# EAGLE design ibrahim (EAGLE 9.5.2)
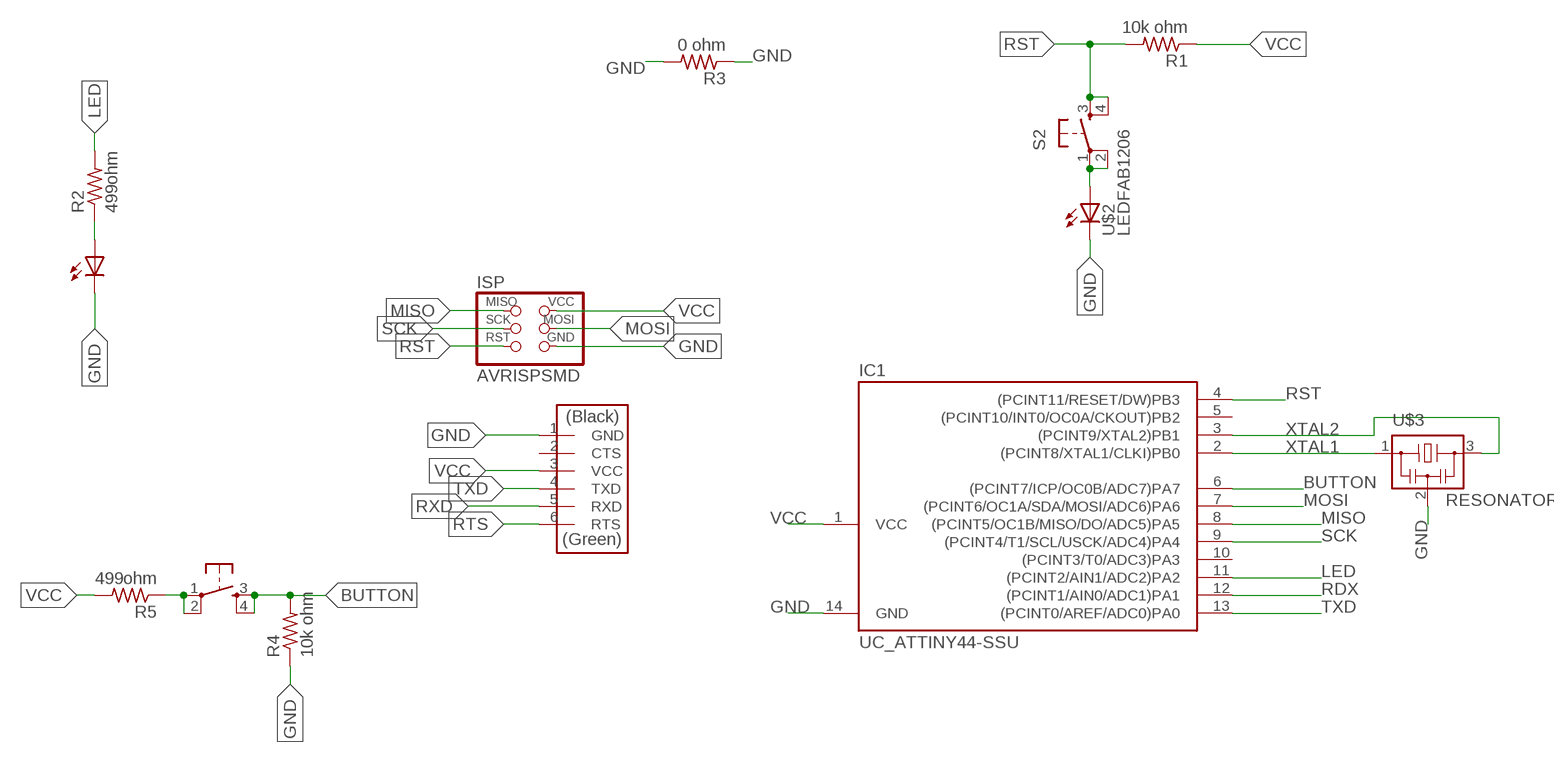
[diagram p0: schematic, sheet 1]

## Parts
IC1  UC_ATTINY44-SSU  [SOIC14]
ISP  AVRISPSMD  [2X03SMD]
R1  10k ohm  R1206FAB  [R1206FAB]
R2  499ohm  R1206FAB  [R1206FAB]
R3  0 ohm  R1206FAB  [R1206FAB]
R4  10k ohm  R1206FAB  [R1206FAB]
R5  499ohm  R1206FAB  [R1206FAB]
S1  6MM_SWITCH6MM_SWITCH  [6MM_SWITCH]
S2  6MM_SWITCH6MM_SWITCH  [6MM_SWITCH]
U$1  FTDI-SMD-HEADER  [1X06SMD]
U$2  LEDFAB1206  [LED1206FAB]
U$3  RESONATOR  [EFOBM]
U$6  LEDFAB1206  [LED1206FAB]

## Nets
BUTTON: IC1.6((PCINT7/ICP/OC0B/ADC7)PA7) R4.2 S1.3(S) S1.4(S1)
GND: IC1.14(GND) ISP.6(GND) R3.1 R3.2 R4.1 U$1.1(GND) U$2.2(C) U$3.2 U$6.2(C)
LED: IC1.11((PCINT2/AIN1/ADC2)PA2) R2.2
MISO: IC1.8((PCINT5/OC1B/MISO/DO/ADC5)PA5) ISP.1(MISO)
MOSI: IC1.7((PCINT6/OC1A/SDA/MOSI/ADC6)PA6) ISP.4(MOSI)
N$1: R2.1 U$6.1(A)
N$2: R5.1 S1.1(P) S1.2(P1)
N$3: S2.1(P) S2.2(P1) U$2.1(A)
RDX: IC1.12((PCINT1/AIN0/ADC1)PA1)
RST: IC1.4((PCINT11/RESET/DW)PB3) ISP.5(RST) R1.2 S2.3(S) S2.4(S1)
RTS: U$1.6(RTS)
RXD: U$1.5(RXD)
SCK: IC1.9((PCINT4/T1/SCL/USCK/ADC4)PA4) ISP.3(SCK)
TXD: IC1.13((PCINT0/AREF/ADC0)PA0) U$1.4(TXD)
VCC: IC1.1(VCC) ISP.2(VCC) R1.1 R5.2 U$1.3(VCC)
XTAL1: IC1.2((PCINT8/XTAL1/CLKI)PB0) U$3.1
XTAL2: IC1.3((PCINT9/XTAL2)PB1) U$3.3
Unconnected: IC1.5((PCINT10/INT0/OC0A/CKOUT)PB2) IC1.10((PCINT3/T0/ADC3)PA3) U$1.2(CTS)

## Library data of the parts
IC1 = fab:UC_ATTINY44
ISP = fab:AVRISP
R1-R5 = fab:R: Resistor (US Symbol)
S1 S2 = fab:6MM_SWITCH: OMRON SWITCH
U$1 = fab:FTDI-SMD-HEADER
U$2 U$6 = fab:LED: LED
U$3 = fab:RESONATOR

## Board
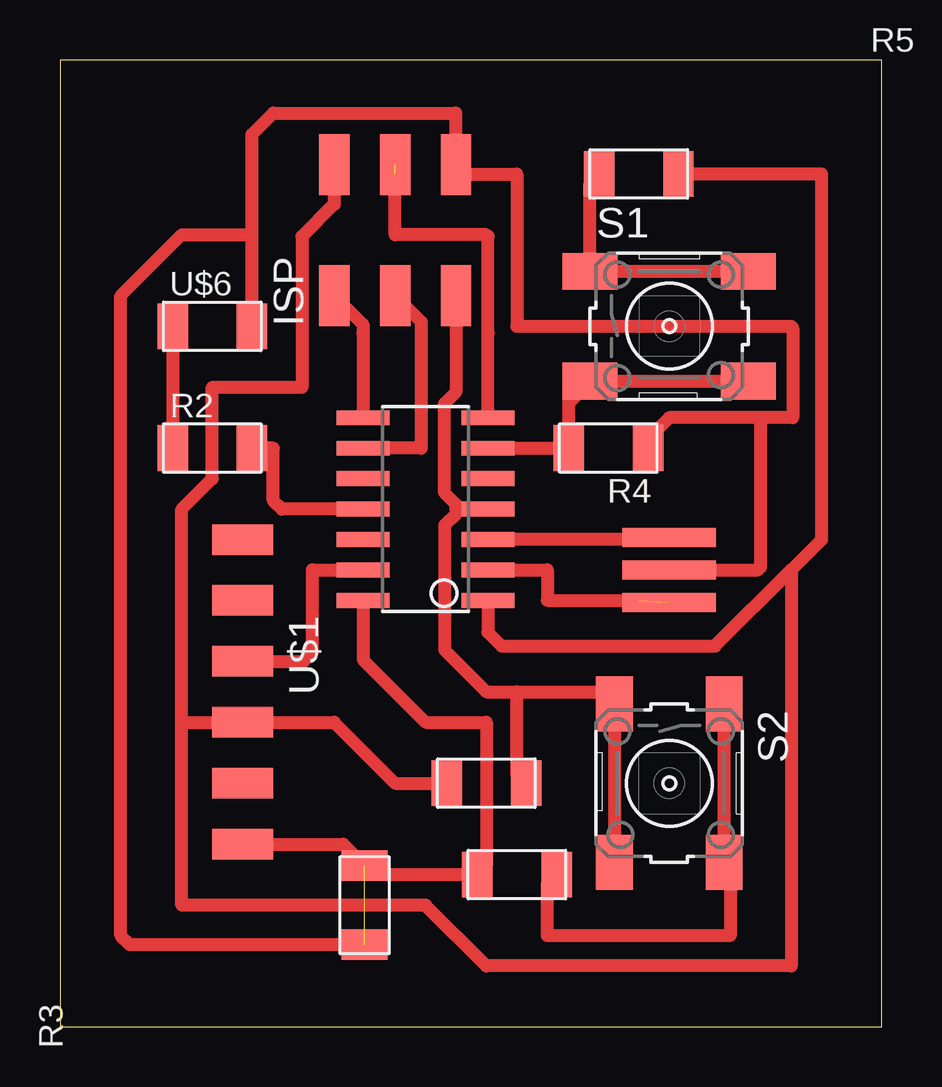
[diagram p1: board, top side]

Size 34.27 x 40.31 mm. Coordinates in mm from the lower left corner, seen from the top.
Outline: 0,0 34.27,0 34.27,40.31 0,40.31 0,0
Copper layers (1*16): Top 0.035mm / dielectric 1.5mm / Bottom 0.035mm
Design rules "default *": minimum track width 0.55mm, minimum drill 0.35mm, track to track 0.43mm, track to pad 0.43mm, pad to pad 0.43mm, via to via 0.43mm, smd to smd 6mil, copper to edge 40mil, drill to drill 6mil, minimum pad ring 10mil, minimum via ring 8mil, stop-mask expansion 4mil, vias tented up to drill 0mil, thermal gap 10mil

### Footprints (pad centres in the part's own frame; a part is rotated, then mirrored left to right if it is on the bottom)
SOIC14 = smd 0.61 x 2.21: 1 -3.81,-2.603; 2 -2.54,-2.603; 3 -1.27,-2.603; 4 0,-2.603; 5 1.27,-2.603; 6 2.54,-2.603; 7 3.81,-2.603; 8 3.81,2.603; 9 2.54,2.603; 10 1.27,2.603; 11 0,2.603; 12 -1.27,2.603; 13 -2.54,2.603; 14 -3.81,2.603
2X03SMD = smd 2.54 x 1.27: 1 -2.54,2.54; 2 2.92,2.54; 3 -2.54,0; 4 2.92,0; 5 -2.54,-2.54; 6 2.92,-2.54
R1206FAB = smd 1.27 x 1.905: 1 -1.651,0; 2 1.651,0
6MM_SWITCH = smd 2.286 x 1.524: 1 -3.302,2.286; 2 3.302,2.286; 3 -3.302,-2.286; 4 3.302,-2.286
1X06SMD = smd 2.54 x 1.27: 1 0,6.35; 2 0,3.81; 3 0,1.27; 4 0,-1.27; 5 0,-3.81; 6 0,-6.35
LED1206FAB = smd 1.27 x 1.905: 1 -1.651,0; 2 1.651,0
EFOBM = smd 0.8 x 3.9: 1 -1.35,0; 2 0,0; 3 1.35,0

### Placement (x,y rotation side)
IC1  15.24,21.59 90 top
ISP  13.97,33.02 90 top
R1  17.78,10.16 0 top
R2  6.35,24.13 0 top
R3  12.7,5.08 90 top
R4  22.86,24.13 180 top
R5  24.13,35.56 0 top
S1  25.4,29.21 0 top
S2  25.4,10.16 270 top
U$1  7.62,13.97 180 top
U$2  19.05,6.35 180 top
U$3  25.4,19.05 90 top
U$6  6.35,29.21 0 top

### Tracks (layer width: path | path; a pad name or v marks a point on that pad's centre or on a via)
BUTTON
  Top 0.55: IC1.6 R4.2 | R4.2 21.59,24.51 | S1.4 S1.3 21.21,26.04 R4.2
GND  (1 unrouted)
  Top 0.55: 29.21,25.4 30.55,25.4 30.55,29.14 30.48,29.21 19.05,29.21 19.05,35.56 16.89,35.56 ISP.6 16.51,38.1 8.89,38.1 8,37.21 8,33.02 | 29.21,25.4 25.4,25.4 24.51,24.51 R4.1 | U$3.2 29.09,19.05 29.21,19.17 29.21,25.4 | 7.62,29.59 U$6.2 8,33.02 | IC1.14 12.64,15.3 15.24,12.7 17.78,12.7 17.78,6.73 U$2.2 13.08,6.35 R3.2 11.81,7.62 U$1.1 | R3.1 2.92,3.43 2.54,3.81 2.54,30.48 5.08,33.02 8,33.02
LED
  Top 0.55: 12.7,21.59 IC1.11 9.25,21.59 8.89,21.95 8.89,24.13 R2.2
MISO
  Top 0.55: ISP.1 12.63,29.28 12.63,28.92 12.64,28.91 IC1.8
MOSI  (1 unrouted)
  Top 0.55: IC1.7 17.84,28.91 17.85,28.92 17.85,32.95 17.78,33.02 13.97,33.02 13.97,35.56
N$1
  Top 0.55: U$6.1 R2.1
N$2
  Top 0.55: S1.2 S1.1 22.1,35.18 R5.1
N$3
  Top 0.55: 28.19,6.35 S2.2 27.94,6.6 27.94,6.35 | 27.94,6.35 27.94,3.81 20.32,3.81 20.32,5.97 U$2.1 | S2.1 27.69,6.6 27.94,6.35
RST
  Top 0.55: IC1.4 16.51,21.59 | S2.3 22.99,13.59 | 16.51,21.59 16.51,21.79 16.03,22.26 16.03,26 16.51,26.47 ISP.5 | 22.86,7.11 S2.4 S2.3 | 16.51,21.59 16.51,21.39 16.03,20.92 16.03,15.72 17.78,13.97 19.05,13.97 | S2.3 22.61,13.97 19.05,13.97 | R1.2 19.05,10.54 19.05,13.97
SCK
  Top 0.55: ISP.3 15.05,29.4 15.05,24.13 IC1.9
TXD
  Top 0.55: IC1.13 10.52,19.05 10.52,15.6 10.16,15.24 U$1.4
VCC
  Top 0.55: 16.51,10.54 R1.1 13.97,10.16 11.43,12.7 U$1.3 5.08,12.7 | IC1.1 17.84,16.45 18.42,15.88 27.3,15.88 30.48,19.05 | R5.2 31.75,35.56 31.75,20.32 30.48,19.05 | ISP.2 11.43,34.29 10.09,32.95 10.09,26.67 6.35,26.67 6.35,22.86 5.08,21.59 5.08,12.7 | 30.48,19.05 30.48,2.54 17.78,2.54 15.24,5.08 5.08,5.08 5.08,12.7
XTAL1  (1 unrouted)
  Top 0.55: IC1.2 20.32,19.05 20.32,17.78 24.13,17.78
XTAL2
  Top 0.55: U$3.3 25.32,20.32 IC1.3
